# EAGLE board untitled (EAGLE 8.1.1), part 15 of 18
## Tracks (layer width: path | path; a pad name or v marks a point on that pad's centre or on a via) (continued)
S$15152 (continued)
  Bottom 0: 49.1,139.71 49.1,139.4
S$15153
  Bottom 0: 49.1,139.4 49.17,139.18
S$15154
  Bottom 0: 146.37,139.57 146.33,139.85
S$15155
  Bottom 0: 146.33,139.85 146.2,140.13
S$15156
  Bottom 0: 146.2,140.13 145.99,140.34
S$15157
  Bottom 0: 145.99,140.34 145.73,140.5
S$15158
  Bottom 0: 145.73,140.5 145.44,140.56
S$15159
  Bottom 0: 145.44,140.56 145.13,140.54
S$15160
  Bottom 0: 145.13,140.54 144.85,140.43
S$15161
  Bottom 0: 144.85,140.43 144.61,140.24
S$15162
  Bottom 0: 144.61,140.24 144.44,140
S$15163
  Bottom 0: 144.44,140 144.36,139.74
S$15164
  Bottom 0: 144.36,139.74 137.85,139.74
S$15165
  Bottom 0: 137.85,139.74 138.05,139.97
S$15166
  Bottom 0: 138.05,139.97 138.19,140.27
S$15167
  Bottom 0: 138.19,140.27 138.24,140.59
S$15168
  Bottom 0: 138.24,140.59 138.19,140.91
S$15169
  Bottom 0: 138.19,140.91 138.05,141.21
S$15170
  Bottom 0: 138.05,141.21 137.84,141.45
S$15171
  Bottom 0: 137.84,141.45 137.66,141.57
S$15172
  Bottom 0: 137.66,141.57 137.66,145.11
S$15173
  Bottom 0: 137.66,145.11 146.76,154.22
S$15174
  Bottom 0: 146.76,154.22 148.03,155.48
S$15175
  Bottom 0: 148.03,155.48 148,155.43
S$15176
  Bottom 0: 148,155.43 147.87,155.01
S$15177
  Bottom 0: 147.87,155.01 147.83,154.56
S$15178
  Bottom 0: 147.83,154.56 147.87,154.11
S$15179
  Bottom 0: 147.87,154.11 148,153.68
S$15180
  Bottom 0: 148,153.68 148.21,153.29
S$15181
  Bottom 0: 148.21,153.29 148.5,152.94
S$15182
  Bottom 0: 148.5,152.94 148.84,152.66
S$15183
  Bottom 0: 148.84,152.66 149.24,152.45
S$15184
  Bottom 0: 149.24,152.45 149.67,152.32
S$15185
  Bottom 0: 149.67,152.32 150.11,152.27
S$15186
  Bottom 0: 150.11,152.27 150.56,152.32
S$15187
  Bottom 0: 150.56,152.32 150.86,152.41
S$15188
  Bottom 0: 150.86,152.41 149.85,151.4
S$15189
  Bottom 0: 149.85,151.4 149.8,151.34
S$15190
  Bottom 0: 149.8,151.34 149.77,151.29
S$15191
  Bottom 0: 149.77,151.29 149.74,151.22
S$15192
  Bottom 0: 149.74,151.22 149.72,151.16
S$15193
  Bottom 0: 149.72,151.16 149.72,151.08
S$15194
  Bottom 0: 149.72,151.08 149.72,148.84
S$15195
  Bottom 0: 149.72,148.84 147.34,146.47
S$15196
  Bottom 0: 147.34,146.47 147.31,146.41
S$15197
  Bottom 0: 147.31,146.41 147.26,146.35
S$15198
  Bottom 0: 147.26,146.35 147.24,146.29
S$15199
  Bottom 0: 147.24,146.29 147.22,146.22
S$15200
  Bottom 0: 147.22,146.22 147.22,146.15
S$15201
  Bottom 0: 147.22,146.15 147.22,140.42
S$15202
  Bottom 0: 147.22,140.42 146.37,139.57
S$15203
  Bottom 0: 139.57,142.66 139.89,142.68
S$15204
  Bottom 0: 139.89,142.68 140.2,142.78
S$15205
  Bottom 0: 140.2,142.78 140.46,142.97
S$15206
  Bottom 0: 140.46,142.97 140.67,143.23
S$15207
  Bottom 0: 140.67,143.23 140.8,143.52
S$15208
  Bottom 0: 140.8,143.52 140.84,143.84
S$15209
  Bottom 0: 140.84,143.84 140.8,144.16
S$15210
  Bottom 0: 140.8,144.16 140.67,144.47
S$15211
  Bottom 0: 140.67,144.47 140.46,144.72
S$15212
  Bottom 0: 140.46,144.72 140.2,144.91
S$15213
  Bottom 0: 140.2,144.91 139.89,145.01
S$15214
  Bottom 0: 139.89,145.01 139.57,145.03
S$15215
  Bottom 0: 139.57,145.03 139.25,144.97
S$15216
  Bottom 0: 139.25,144.97 138.96,144.82
S$15217
  Bottom 0: 138.96,144.82 138.72,144.6
S$15218
  Bottom 0: 138.72,144.6 138.55,144.32
S$15219
  Bottom 0: 138.55,144.32 138.47,144.01
S$15220
  Bottom 0: 138.47,144.01 138.47,143.68
S$15221
  Bottom 0: 138.47,143.68 138.55,143.37
S$15222
  Bottom 0: 138.55,143.37 138.72,143.09
S$15223
  Bottom 0: 138.72,143.09 138.96,142.87
S$15224
  Bottom 0: 138.96,142.87 139.25,142.72
S$15225
  Bottom 0: 139.25,142.72 139.57,142.66
S$15226
  Bottom 0: 147.66,148.09 148.01,148.15
S$15227
  Bottom 0: 148.01,148.15 148.32,148.3
S$15228
  Bottom 0: 148.32,148.3 148.59,148.52
S$15229
  Bottom 0: 148.59,148.52 148.8,148.81
S$15230
  Bottom 0: 148.8,148.81 148.93,149.13
S$15231
  Bottom 0: 148.93,149.13 148.97,149.48
S$15232
  Bottom 0: 148.97,149.48 148.93,149.82
S$15233
  Bottom 0: 148.93,149.82 148.8,150.15
S$15234
  Bottom 0: 148.8,150.15 148.59,150.43
S$15235
  Bottom 0: 148.59,150.43 148.32,150.66
S$15236
  Bottom 0: 148.32,150.66 148.01,150.81
S$15237
  Bottom 0: 148.01,150.81 147.66,150.87
S$15238
  Bottom 0: 147.66,150.87 147.31,150.85
S$15239
  Bottom 0: 147.31,150.85 146.98,150.74
S$15240
  Bottom 0: 146.98,150.74 146.69,150.56
S$15241
  Bottom 0: 146.69,150.56 146.44,150.3
S$15242
  Bottom 0: 146.44,150.3 146.27,149.99
S$15243
  Bottom 0: 146.27,149.99 146.19,149.65
S$15244
  Bottom 0: 146.19,149.65 146.19,149.3
S$15245
  Bottom 0: 146.19,149.3 146.27,148.97
S$15246
  Bottom 0: 146.27,148.97 146.44,148.66
S$15247
  Bottom 0: 146.44,148.66 146.69,148.4
S$15248
  Bottom 0: 146.69,148.4 146.98,148.21
S$15249
  Bottom 0: 146.98,148.21 147.31,148.11
S$15250
  Bottom 0: 147.31,148.11 147.66,148.09
S$15251
  Bottom 0: 59.5,139.69 59.5,141.48
S$15252
  Bottom 0: 59.5,141.48 59.49,141.55
S$15253
  Bottom 0: 59.49,141.55 59.45,141.62
S$15254
  Bottom 0: 59.45,141.62 59.4,141.68
S$15255
  Bottom 0: 59.4,141.68 59.32,141.72
S$15256
  Bottom 0: 59.32,141.72 59.25,141.73
S$15257
  Bottom 0: 59.25,141.73 58.8,141.73
S$15258
  Bottom 0: 58.8,141.73 58.8,141.86
S$15259
  Bottom 0: 58.8,141.86 58.74,142.08
S$15260
  Bottom 0: 58.74,142.08 58.58,142.24
S$15261
  Bottom 0: 58.58,142.24 58.36,142.3
S$15262
  Bottom 0: 58.36,142.3 57.99,142.3
S$15263
  Bottom 0: 57.99,142.3 56.91,143.38
S$15264
  Bottom 0: 56.91,143.38 56.97,143.52
S$15265
  Bottom 0: 56.97,143.52 57.02,143.84
S$15266
  Bottom 0: 57.02,143.84 56.97,144.16
S$15267
  Bottom 0: 56.97,144.16 56.84,144.46
S$15268
  Bottom 0: 56.84,144.46 56.64,144.71
S$15269
  Bottom 0: 56.64,144.71 56.57,144.76
S$15270
  Bottom 0: 56.57,144.76 61.72,144.76
S$15271
  Bottom 0: 61.72,144.76 62.3,144.18
S$15272
  Bottom 0: 62.3,144.18 62.26,144
S$15273
  Bottom 0: 62.26,144 62.26,143.68
S$15274
  Bottom 0: 62.26,143.68 62.35,143.36
S$15275
  Bottom 0: 62.35,143.36 62.52,143.09
S$15276
  Bottom 0: 62.52,143.09 62.75,142.87
S$15277
  Bottom 0: 62.75,142.87 63.04,142.72
S$15278
  Bottom 0: 63.04,142.72 63.36,142.65
S$15279
  Bottom 0: 63.36,142.65 63.69,142.67
S$15280
  Bottom 0: 63.69,142.67 63.99,142.78
S$15281
  Bottom 0: 63.99,142.78 64.26,142.97
S$15282
  Bottom 0: 64.26,142.97 64.46,143.22
S$15283
  Bottom 0: 64.46,143.22 64.49,143.27
S$15284
  Bottom 0: 64.49,143.27 66.41,143.27
S$15285
  Bottom 0: 66.41,143.27 69.13,140.56
S$15286
  Bottom 0: 69.13,140.56 68.92,140.54
S$15287
  Bottom 0: 68.92,140.54 68.65,140.43
S$15288
  Bottom 0: 68.65,140.43 68.41,140.24
S$15289
  Bottom 0: 68.41,140.24 68.24,140
S$15290
  Bottom 0: 68.24,140 68.15,139.71
S$15291
  Bottom 0: 68.15,139.71 68.15,139.69
S$15292
  Bottom 0: 68.15,139.69 61.59,139.69
S$15293
  Bottom 0: 61.59,139.69 61.65,139.72
S$15294
  Bottom 0: 61.65,139.72 61.86,139.97
S$15295
  Bottom 0: 61.86,139.97 62,140.27
S$15296
  Bottom 0: 62,140.27 62.04,140.59
S$15297
  Bottom 0: 62.04,140.59 62,140.91
S$15298
  Bottom 0: 62,140.91 61.86,141.21
S$15299
  Bottom 0: 61.86,141.21 61.65,141.45
S$15300
  Bottom 0: 61.65,141.45 61.37,141.63
S$15301
  Bottom 0: 61.37,141.63 61.06,141.72
S$15302
  Bottom 0: 61.06,141.72 60.74,141.72
S$15303
  Bottom 0: 60.74,141.72 60.42,141.63
S$15304
  Bottom 0: 60.42,141.63 60.15,141.45
S$15305
  Bottom 0: 60.15,141.45 59.94,141.21
S$15306
  Bottom 0: 59.94,141.21 59.8,140.91
S$15307
  Bottom 0: 59.8,140.91 59.76,140.59
S$15308
  Bottom 0: 59.76,140.59 59.8,140.27
S$15309
  Bottom 0: 59.8,140.27 59.94,139.97
S$15310
  Bottom 0: 59.94,139.97 60.15,139.72
S$15311
  Bottom 0: 60.15,139.72 60.21,139.69
S$15312
  Bottom 0: 60.21,139.69 59.5,139.69
S$15313
  Bottom 0: 154.75,140 154.75,141.48
S$15314
  Bottom 0: 154.75,141.48 154.74,141.55
S$15315
  Bottom 0: 154.74,141.55 154.7,141.62
S$15316
  Bottom 0: 154.7,141.62 154.64,141.68
S$15317
  Bottom 0: 154.64,141.68 154.57,141.72
S$15318
  Bottom 0: 154.57,141.72 154.49,141.73
S$15319
  Bottom 0: 154.49,141.73 154.05,141.73
S$15320
  Bottom 0: 154.05,141.73 154.05,141.86
S$15321
  Bottom 0: 154.05,141.86 153.99,142.08
S$15322
  Bottom 0: 153.99,142.08 153.82,142.24
S$15323
  Bottom 0: 153.82,142.24 153.6,142.3
S$15324
  Bottom 0: 153.6,142.3 153.26,142.3
S$15325
  Bottom 0: 153.26,142.3 152.17,143.39
S$15326
  Bottom 0: 152.17,143.39 152.23,143.52
S$15327
  Bottom 0: 152.23,143.52 152.28,143.84
S$15328
  Bottom 0: 152.28,143.84 152.23,144.16
S$15329
  Bottom 0: 152.23,144.16 152.1,144.47
S$15330
  Bottom 0: 152.1,144.47 151.9,144.72
S$15331
  Bottom 0: 151.9,144.72 151.63,144.91
S$15332
  Bottom 0: 151.63,144.91 151.33,145.01
S$15333
  Bottom 0: 151.33,145.01 151,145.03
S$15334
  Bottom 0: 151,145.03 150.92,145.02
S$15335
  Bottom 0: 150.92,145.02 157.26,151.36
S$15336
  Bottom 0: 157.26,151.36 157.66,151.36
S$15337
  Bottom 0: 157.66,151.36 157.73,151.36
S$15338
  Bottom 0: 157.73,151.36 157.79,151.38
S$15339
  Bottom 0: 157.79,151.38 157.86,151.4
S$15340
  Bottom 0: 157.86,151.4 157.92,151.44
S$15341
  Bottom 0: 157.92,151.44 157.97,151.49
S$15342
  Bottom 0: 157.97,151.49 158.18,151.68
S$15343
  Bottom 0: 158.18,151.68 158.21,151.68
S$15344
  Bottom 0: 158.21,151.68 158.28,151.67
S$15345
  Bottom 0: 158.28,151.67 158.91,151.67
S$15346
  Bottom 0: 158.91,151.67 158.74,151.43
S$15347
  Bottom 0: 158.74,151.43 158.65,151.13
S$15348
  Bottom 0: 158.65,151.13 158.65,150.83
S$15349
  Bottom 0: 158.65,150.83 158.74,150.54
S$15350
  Bottom 0: 158.74,150.54 158.91,150.29
S$15351
  Bottom 0: 158.91,150.29 159.14,150.1
S$15352
  Bottom 0: 159.14,150.1 159.43,149.99
S$15353
  Bottom 0: 159.43,149.99 159.73,149.97
S$15354
  Bottom 0: 159.73,149.97 160.03,150.04
S$15355
  Bottom 0: 160.03,150.04 160.29,150.19
S$15356
  Bottom 0: 160.29,150.19 160.49,150.41
S$15357
  Bottom 0: 160.49,150.41 160.62,150.68
S$15358
  Bottom 0: 160.62,150.68 160.67,150.98
S$15359
  Bottom 0: 160.67,150.98 160.62,151.28
S$15360
  Bottom 0: 160.62,151.28 160.49,151.56
S$15361
  Bottom 0: 160.49,151.56 160.39,151.67
S$15362
  Bottom 0: 160.39,151.67 170.46,151.67
S$15363
  Bottom 0: 170.46,151.67 170.53,151.68
S$15364
  Bottom 0: 170.53,151.68 170.6,151.69
S$15365
  Bottom 0: 170.6,151.69 170.66,151.72
S$15366
  Bottom 0: 170.66,151.72 170.72,151.76
S$15367
  Bottom 0: 170.72,151.76 170.77,151.8
S$15368
  Bottom 0: 170.77,151.8 172.09,153.12
S$15369
  Bottom 0: 172.09,153.12 172.13,153.12
S$15370
  Bottom 0: 172.13,153.12 172.09,153.1
S$15371
  Bottom 0: 172.09,153.1 171.85,152.84
S$15372
  Bottom 0: 171.85,152.84 171.67,152.53
S$15373
  Bottom 0: 171.67,152.53 171.59,152.19
S$15374
  Bottom 0: 171.59,152.19 171.59,151.84
S$15375
  Bottom 0: 171.59,151.84 171.67,151.51
S$15376
  Bottom 0: 171.67,151.51 171.73,151.4
S$15377
  Bottom 0: 171.73,151.4 168.6,148.28
S$15378
  Bottom 0: 168.6,148.28 167.33,148.28
S$15379
  Bottom 0: 167.33,148.28 167.37,148.3
S$15380
  Bottom 0: 167.37,148.3 167.64,148.52
S$15381
  Bottom 0: 167.64,148.52 167.85,148.81
S$15382
  Bottom 0: 167.85,148.81 167.97,149.13
S$15383
  Bottom 0: 167.97,149.13 168.02,149.48
S$15384
  Bottom 0: 168.02,149.48 167.97,149.82
S$15385
  Bottom 0: 167.97,149.82 167.85,150.15
S$15386
  Bottom 0: 167.85,150.15 167.64,150.43
S$15387
  Bottom 0: 167.64,150.43 167.37,150.66
S$15388
  Bottom 0: 167.37,150.66 167.06,150.81
S$15389
  Bottom 0: 167.06,150.81 166.71,150.87
S$15390
  Bottom 0: 166.71,150.87 166.36,150.85
S$15391
  Bottom 0: 166.36,150.85 166.03,150.74
S$15392
  Bottom 0: 166.03,150.74 165.74,150.56
S$15393
  Bottom 0: 165.74,150.56 165.49,150.3
S$15394
  Bottom 0: 165.49,150.3 165.32,149.99
S$15395
  Bottom 0: 165.32,149.99 165.24,149.65
S$15396
  Bottom 0: 165.24,149.65 165.24,149.3
S$15397
  Bottom 0: 165.24,149.3 165.32,148.97
S$15398
  Bottom 0: 165.32,148.97 165.49,148.66
S$15399
  Bottom 0: 165.49,148.66 165.74,148.4
S$15400
  Bottom 0: 165.74,148.4 165.93,148.28
S$15401
  Bottom 0: 165.93,148.28 155.93,148.28
S$15402
  Bottom 0: 155.93,148.28 155.86,148.28
S$15403
  Bottom 0: 155.86,148.28 155.79,148.26
S$15404
  Bottom 0: 155.79,148.26 155.73,148.23
S$15405
  Bottom 0: 155.73,148.23 155.67,148.19
S$15406
  Bottom 0: 155.67,148.19 155.62,148.15
S$15407
  Bottom 0: 155.62,148.15 153.85,146.39
S$15408
  Bottom 0: 153.85,146.39 153.81,146.33
S$15409
  Bottom 0: 153.81,146.33 153.77,146.28
S$15410
  Bottom 0: 153.77,146.28 153.74,146.21
S$15411
  Bottom 0: 153.74,146.21 153.73,146.15
S$15412
  Bottom 0: 153.73,146.15 153.72,146.07
S$15413
  Bottom 0: 153.72,146.07 153.72,144.78
S$15414
  Bottom 0: 153.72,144.78 153.73,144.71
S$15415
  Bottom 0: 153.73,144.71 153.74,144.64
S$15416
  Bottom 0: 153.74,144.64 153.77,144.58
S$15417
  Bottom 0: 153.77,144.58 153.81,144.52
S$15418
  Bottom 0: 153.81,144.52 153.85,144.47
S$15419
  Bottom 0: 153.85,144.47 156.8,141.51
S$15420
  Bottom 0: 156.8,141.51 156.62,141.63
S$15421
  Bottom 0: 156.62,141.63 156.31,141.72
S$15422
  Bottom 0: 156.31,141.72 155.98,141.72
S$15423
  Bottom 0: 155.98,141.72 155.67,141.63
S$15424
  Bottom 0: 155.67,141.63 155.4,141.45
S$15425
  Bottom 0: 155.4,141.45 155.18,141.21
S$15426
  Bottom 0: 155.18,141.21 155.04,140.91
S$15427
  Bottom 0: 155.04,140.91 155,140.59
S$15428
  Bottom 0: 155,140.59 155.04,140.29
S$15429
  Bottom 0: 155.04,140.29 154.75,140
S$15430
  Bottom 0: 240.79,142.26 240.78,142.27
S$15431
  Bottom 0: 240.78,142.27 240.72,142.29
S$15432
  Bottom 0: 240.72,142.29 240.65,142.29
S$15433
  Bottom 0: 240.65,142.29 223.56,142.29
S$15434
  Bottom 0: 223.56,142.29 207.94,157.9
S$15435
  Bottom 0: 207.94,157.9 211.02,157.9
S$15436
  Bottom 0: 211.02,157.9 216.95,151.98
S$15437
  Bottom 0: 216.95,151.98 216.88,151.99
S$15438
  Bottom 0: 216.88,151.99 216.58,151.97
S$15439
  Bottom 0: 216.58,151.97 216.3,151.86
S$15440
  Bottom 0: 216.3,151.86 216.06,151.67
S$15441
  Bottom 0: 216.06,151.67 215.89,151.43
S$15442
  Bottom 0: 215.89,151.43 215.8,151.13
S$15443
  Bottom 0: 215.8,151.13 215.8,150.83
S$15444
  Bottom 0: 215.8,150.83 215.89,150.54
S$15445
  Bottom 0: 215.89,150.54 216.06,150.29
S$15446
  Bottom 0: 216.06,150.29 216.3,150.1
S$15447
  Bottom 0: 216.3,150.1 216.58,149.99
S$15448
  Bottom 0: 216.58,149.99 216.88,149.97
S$15449
  Bottom 0: 216.88,149.97 217.18,150.04
S$15450
  Bottom 0: 217.18,150.04 217.44,150.19
S$15451
  Bottom 0: 217.44,150.19 217.64,150.41
S$15452
  Bottom 0: 217.64,150.41 217.71,150.54
S$15453
  Bottom 0: 217.71,150.54 222.08,150.54
S$15454
  Bottom 0: 222.08,150.54 222.53,150.09
S$15455
  Bottom 0: 222.53,150.09 222.47,149.99
S$15456
  Bottom 0: 222.47,149.99 222.39,149.65
S$15457
  Bottom 0: 222.39,149.65 222.39,149.3
S$15458
  Bottom 0: 222.39,149.3 222.47,148.97
S$15459
  Bottom 0: 222.47,148.97 222.65,148.66
S$15460
  Bottom 0: 222.65,148.66 222.88,148.4
S$15461
  Bottom 0: 222.88,148.4 223.18,148.21
S$15462
  Bottom 0: 223.18,148.21 223.51,148.11
S$15463
  Bottom 0: 223.51,148.11 223.86,148.09
S$15464
  Bottom 0: 223.86,148.09 224.21,148.15
S$15465
  Bottom 0: 224.21,148.15 224.52,148.3
S$15466
  Bottom 0: 224.52,148.3 224.79,148.52
S$15467
  Bottom 0: 224.79,148.52 225,148.81
S$15468
  Bottom 0: 225,148.81 225.12,149.13
S$15469
  Bottom 0: 225.12,149.13 225.17,149.48
S$15470
  Bottom 0: 225.17,149.48 225.12,149.82
S$15471
  Bottom 0: 225.12,149.82 225,150.15
S$15472
  Bottom 0: 225,150.15 224.79,150.43
S$15473
  Bottom 0: 224.79,150.43 224.52,150.66
S$15474
  Bottom 0: 224.52,150.66 224.21,150.81
S$15475
  Bottom 0: 224.21,150.81 223.86,150.87
S$15476
  Bottom 0: 223.86,150.87 223.51,150.85
S$15477
  Bottom 0: 223.51,150.85 223.18,150.74
S$15478
  Bottom 0: 223.18,150.74 223.15,150.72
S$15479
  Bottom 0: 223.15,150.72 222.57,151.3
S$15480
  Bottom 0: 222.57,151.3 222.52,151.34
S$15481
  Bottom 0: 222.52,151.34 222.46,151.38
S$15482
  Bottom 0: 222.46,151.38 222.4,151.4
S$15483
  Bottom 0: 222.4,151.4 222.33,151.42
S$15484
  Bottom 0: 222.33,151.42 222.26,151.43
S$15485
  Bottom 0: 222.26,151.43 217.71,151.43
S$15486
  Bottom 0: 217.71,151.43 217.64,151.56
S$15487
  Bottom 0: 217.64,151.56 217.62,151.58
S$15488
  Bottom 0: 217.62,151.58 228.8,151.58
S$15489
  Bottom 0: 228.8,151.58 228.82,151.51
S$15490
  Bottom 0: 228.82,151.51 229,151.2
S$15491
  Bottom 0: 229,151.2 229.24,150.94
S$15492
  Bottom 0: 229.24,150.94 229.53,150.75
S$15493
  Bottom 0: 229.53,150.75 229.86,150.65
S$15494
  Bottom 0: 229.86,150.65 230.21,150.63
S$15495
  Bottom 0: 230.21,150.63 230.56,150.69
S$15496
  Bottom 0: 230.56,150.69 230.87,150.84
S$15497
  Bottom 0: 230.87,150.84 231.14,151.06
S$15498
  Bottom 0: 231.14,151.06 231.35,151.35
S$15499
  Bottom 0: 231.35,151.35 231.44,151.58
S$15500
  Bottom 0: 231.44,151.58 231.48,151.58
S$15501
  Bottom 0: 231.48,151.58 240.79,142.26
S$15502
  Bottom 0: 227.21,142.65 227.53,142.67
S$15503
  Bottom 0: 227.53,142.67 227.84,142.78
S$15504
  Bottom 0: 227.84,142.78 228.1,142.97
S$15505
  Bottom 0: 228.1,142.97 228.31,143.22
S$15506
  Bottom 0: 228.31,143.22 228.44,143.52
S$15507
  Bottom 0: 228.44,143.52 228.48,143.84
S$15508
  Bottom 0: 228.48,143.84 228.44,144.16
S$15509
  Bottom 0: 228.44,144.16 228.31,144.46
S$15510
  Bottom 0: 228.31,144.46 228.1,144.71
S$15511
  Bottom 0: 228.1,144.71 227.84,144.9
S$15512
  Bottom 0: 227.84,144.9 227.53,145.01
S$15513
  Bottom 0: 227.53,145.01 227.21,145.03
S$15514
  Bottom 0: 227.21,145.03 226.89,144.96
S$15515
  Bottom 0: 226.89,144.96 226.6,144.82
S$15516
  Bottom 0: 226.6,144.82 226.37,144.59
S$15517
  Bottom 0: 226.37,144.59 226.19,144.32
S$15518
  Bottom 0: 226.19,144.32 226.11,144
S$15519
  Bottom 0: 226.11,144 226.11,143.68
S$15520
  Bottom 0: 226.11,143.68 226.19,143.36
S$15521
  Bottom 0: 226.19,143.36 226.37,143.09
S$15522
  Bottom 0: 226.37,143.09 226.6,142.87
S$15523
  Bottom 0: 226.6,142.87 226.89,142.72
S$15524
  Bottom 0: 226.89,142.72 227.21,142.65
S$15525
  Bottom 0: 234.83,142.65 235.15,142.67
S$15526
  Bottom 0: 235.15,142.67 235.46,142.78
S$15527
  Bottom 0: 235.46,142.78 235.72,142.97
S$15528
  Bottom 0: 235.72,142.97 235.93,143.22
S$15529
  Bottom 0: 235.93,143.22 236.06,143.52
S$15530
  Bottom 0: 236.06,143.52 236.1,143.84
S$15531
  Bottom 0: 236.1,143.84 236.06,144.16
S$15532
  Bottom 0: 236.06,144.16 235.93,144.46
S$15533
  Bottom 0: 235.93,144.46 235.72,144.71
S$15534
  Bottom 0: 235.72,144.71 235.46,144.9
S$15535
  Bottom 0: 235.46,144.9 235.15,145.01
S$15536
  Bottom 0: 235.15,145.01 234.83,145.03
S$15537
  Bottom 0: 234.83,145.03 234.51,144.96
S$15538
  Bottom 0: 234.51,144.96 234.22,144.82
S$15539
  Bottom 0: 234.22,144.82 233.99,144.59
S$15540
  Bottom 0: 233.99,144.59 233.81,144.32
S$15541
  Bottom 0: 233.81,144.32 233.73,144
S$15542
  Bottom 0: 233.73,144 233.73,143.68
S$15543
  Bottom 0: 233.73,143.68 233.81,143.36
S$15544
  Bottom 0: 233.81,143.36 233.99,143.09
S$15545
  Bottom 0: 233.99,143.09 234.22,142.87
S$15546
  Bottom 0: 234.22,142.87 234.51,142.72
S$15547
  Bottom 0: 234.51,142.72 234.83,142.65
S$15548
  Bottom 0: 103.41,142.78 102.69,143.5
S$15549
  Bottom 0: 102.69,143.5 102.69,143.52
S$15550
  Bottom 0: 102.69,143.52 102.74,143.84
S$15551
  Bottom 0: 102.74,143.84 102.69,144.16
S$15552
  Bottom 0: 102.69,144.16 102.69,144.18
S$15553
  Bottom 0: 102.69,144.18 104.18,145.67
S$15554
  Bottom 0: 104.18,145.67 104.24,145.74
S$15555
  Bottom 0: 104.24,145.74 104.28,145.81
S$15556
  Bottom 0: 104.28,145.81 104.32,145.89
S$15557
  Bottom 0: 104.32,145.89 104.34,145.98
S$15558
  Bottom 0: 104.34,145.98 104.34,146.07
S$15559
  Bottom 0: 104.34,146.07 104.34,162.5
S$15560
  Bottom 0: 104.34,162.5 104.65,162.8
S$15561
  Bottom 0: 104.65,162.8 104.65,162.75
S$15562
  Bottom 0: 104.65,162.75 104.74,162.52
S$15563
  Bottom 0: 104.74,162.52 104.91,162.33
S$15564
  Bottom 0: 104.91,162.33 105.13,162.22
S$15565
  Bottom 0: 105.13,162.22 105.16,162.22
S$15566
  Bottom 0: 105.16,162.22 109.98,157.4
S$15567
  Bottom 0: 109.98,157.4 110.04,157.36
S$15568
  Bottom 0: 110.04,157.36 110.1,157.32
S$15569
  Bottom 0: 110.1,157.32 110.16,157.29
S$15570
  Bottom 0: 110.16,157.29 110.23,157.28
S$15571
  Bottom 0: 110.23,157.28 110.3,157.27
S$15572
  Bottom 0: 110.3,157.27 112.2,157.27
S$15573
  Bottom 0: 112.2,157.27 112.76,156.71
S$15574
  Bottom 0: 112.76,156.71 112.46,156.8
S$15575
  Bottom 0: 112.46,156.8 112.01,156.84
S$15576
  Bottom 0: 112.01,156.84 111.57,156.8
S$15577
  Bottom 0: 111.57,156.8 111.14,156.67
S$15578
  Bottom 0: 111.14,156.67 110.74,156.46
S$15579
  Bottom 0: 110.74,156.46 110.4,156.17
S$15580
  Bottom 0: 110.4,156.17 110.11,155.83
S$15581
  Bottom 0: 110.11,155.83 109.9,155.43
S$15582
  Bottom 0: 109.9,155.43 109.77,155.01
S$15583
  Bottom 0: 109.77,155.01 109.73,154.56
S$15584
  Bottom 0: 109.73,154.56 109.77,154.11
S$15585
  Bottom 0: 109.77,154.11 109.9,153.68
S$15586
  Bottom 0: 109.9,153.68 110.11,153.29
S$15587
  Bottom 0: 110.11,153.29 110.4,152.94
S$15588
  Bottom 0: 110.4,152.94 110.74,152.66
S$15589
  Bottom 0: 110.74,152.66 111.14,152.45
S$15590
  Bottom 0: 111.14,152.45 111.57,152.32
S$15591
  Bottom 0: 111.57,152.32 112.01,152.27
S$15592
  Bottom 0: 112.01,152.27 112.46,152.32
S$15593
  Bottom 0: 112.46,152.32 112.89,152.45
S$15594
  Bottom 0: 112.89,152.45 113.28,152.66
S$15595
  Bottom 0: 113.28,152.66 113.63,152.94
S$15596
  Bottom 0: 113.63,152.94 113.91,153.29
S$15597
  Bottom 0: 113.91,153.29 114.13,153.68
S$15598
  Bottom 0: 114.13,153.68 114.25,154.11
S$15599
  Bottom 0: 114.25,154.11 114.3,154.56
S$15600
  Bottom 0: 114.3,154.56 114.25,155.01
S$15601
  Bottom 0: 114.25,155.01 114.16,155.31
S$15602
  Bottom 0: 114.16,155.31 115.38,154.09
S$15603
  Bottom 0: 115.38,154.09 115.38,153.34
S$15604
  Bottom 0: 115.38,153.34 115.23,153.28
S$15605
  Bottom 0: 115.23,153.28 114.94,153.1
S$15606
  Bottom 0: 114.94,153.1 114.69,152.84
S$15607
  Bottom 0: 114.69,152.84 114.52,152.53
S$15608
  Bottom 0: 114.52,152.53 114.44,152.19
S$15609
  Bottom 0: 114.44,152.19 114.44,151.84
S$15610
  Bottom 0: 114.44,151.84 114.52,151.51
S$15611
  Bottom 0: 114.52,151.51 114.69,151.2
S$15612
  Bottom 0: 114.69,151.2 114.94,150.94
S$15613
  Bottom 0: 114.94,150.94 115.23,150.75
S$15614
  Bottom 0: 115.23,150.75 115.56,150.65
S$15615
  Bottom 0: 115.56,150.65 115.91,150.63
S$15616
  Bottom 0: 115.91,150.63 116.26,150.69
S$15617
  Bottom 0: 116.26,150.69 116.44,150.78
S$15618
  Bottom 0: 116.44,150.78 121.51,145.7
S$15619
  Bottom 0: 121.51,145.7 121.51,144.6
S$15620
  Bottom 0: 121.51,144.6 121.41,144.72
S$15621
  Bottom 0: 121.41,144.72 121.15,144.91
S$15622
  Bottom 0: 121.15,144.91 120.84,145.01
S$15623
  Bottom 0: 120.84,145.01 120.52,145.03
S$15624
  Bottom 0: 120.52,145.03 120.2,144.97
S$15625
  Bottom 0: 120.2,144.97 119.91,144.82
S$15626
  Bottom 0: 119.91,144.82 119.67,144.6
S$15627
  Bottom 0: 119.67,144.6 119.5,144.32
S$15628
  Bottom 0: 119.5,144.32 119.42,144.01
S$15629
  Bottom 0: 119.42,144.01 119.42,143.68
S$15630
  Bottom 0: 119.42,143.68 119.46,143.51
S$15631
  Bottom 0: 119.46,143.51 118.72,142.78
S$15632
  Bottom 0: 118.72,142.78 113.51,142.78
S$15633
  Bottom 0: 113.51,142.78 113.53,142.78
S$15634
  Bottom 0: 113.53,142.78 113.79,142.97
S$15635
  Bottom 0: 113.79,142.97 114,143.23
S$15636
  Bottom 0: 114,143.23 114.13,143.52
S$15637
  Bottom 0: 114.13,143.52 114.17,143.84
S$15638
  Bottom 0: 114.17,143.84 114.13,144.16
S$15639
  Bottom 0: 114.13,144.16 114,144.47
S$15640
  Bottom 0: 114,144.47 113.79,144.72
S$15641
  Bottom 0: 113.79,144.72 113.53,144.91
S$15642
  Bottom 0: 113.53,144.91 113.22,145.01
S$15643
  Bottom 0: 113.22,145.01 112.9,145.03
S$15644
  Bottom 0: 112.9,145.03 112.58,144.97
S$15645
  Bottom 0: 112.58,144.97 112.29,144.82
S$15646
  Bottom 0: 112.29,144.82 112.06,144.6
S$15647
  Bottom 0: 112.06,144.6 111.88,144.32
S$15648
  Bottom 0: 111.88,144.32 111.8,144.01
S$15649
  Bottom 0: 111.8,144.01 111.8,143.68
S$15650
  Bottom 0: 111.8,143.68 111.88,143.37
S$15651
  Bottom 0: 111.88,143.37 112.06,143.09
S$15652
  Bottom 0: 112.06,143.09 112.29,142.87
S$15653
  Bottom 0: 112.29,142.87 112.47,142.78
S$15654
  Bottom 0: 112.47,142.78 103.41,142.78
S$15655
  Bottom 0: 109.56,148.09 109.91,148.15
S$15656
  Bottom 0: 109.91,148.15 110.22,148.3
S$15657
  Bottom 0: 110.22,148.3 110.49,148.52
S$15658
  Bottom 0: 110.49,148.52 110.7,148.81
S$15659
  Bottom 0: 110.7,148.81 110.83,149.13
S$15660
  Bottom 0: 110.83,149.13 110.87,149.48
S$15661
  Bottom 0: 110.87,149.48 110.83,149.82
S$15662
  Bottom 0: 110.83,149.82 110.7,150.15
S$15663
  Bottom 0: 110.7,150.15 110.49,150.43
S$15664
  Bottom 0: 110.49,150.43 110.22,150.66
S$15665
  Bottom 0: 110.22,150.66 109.91,150.81
S$15666
  Bottom 0: 109.91,150.81 109.56,150.87
S$15667
  Bottom 0: 109.56,150.87 109.21,150.85
S$15668
  Bottom 0: 109.21,150.85 108.88,150.74
S$15669
  Bottom 0: 108.88,150.74 108.58,150.56
S$15670
  Bottom 0: 108.58,150.56 108.34,150.3
S$15671
  Bottom 0: 108.34,150.3 108.17,149.99
S$15672
  Bottom 0: 108.17,149.99 108.09,149.65
S$15673
  Bottom 0: 108.09,149.65 108.09,149.3
S$15674
  Bottom 0: 108.09,149.3 108.17,148.97
S$15675
  Bottom 0: 108.17,148.97 108.34,148.66
S$15676
  Bottom 0: 108.34,148.66 108.58,148.4
S$15677
  Bottom 0: 108.58,148.4 108.88,148.21
S$15678
  Bottom 0: 108.88,148.21 109.21,148.11
S$15679
  Bottom 0: 109.21,148.11 109.56,148.09
S$15680
  Bottom 0: 261.74,142.83 258.56,146.01
S$15681
  Bottom 0: 258.56,146.01 258.55,146.02
S$15682
  Bottom 0: 258.55,146.02 253.27,151.3
S$15683
  Bottom 0: 253.27,151.3 253.22,151.35
S$15684
  Bottom 0: 253.22,151.35 253.16,151.39
S$15685
  Bottom 0: 253.16,151.39 253.1,151.41
S$15686
  Bottom 0: 253.1,151.41 253.03,151.43
S$15687
  Bottom 0: 253.03,151.43 252.96,151.44
S$15688
  Bottom 0: 252.96,151.44 250.43,151.44
S$15689
  Bottom 0: 250.43,151.44 250.53,151.67
S$15690
  Bottom 0: 250.53,151.67 250.57,152.02
S$15691
  Bottom 0: 250.57,152.02 250.53,152.36
S$15692
  Bottom 0: 250.53,152.36 250.4,152.69
S$15693
  Bottom 0: 250.4,152.69 250.19,152.97
S$15694
  Bottom 0: 250.19,152.97 249.92,153.2
S$15695
  Bottom 0: 249.92,153.2 249.61,153.35
S$15696
  Bottom 0: 249.61,153.35 249.26,153.41
S$15697
  Bottom 0: 249.26,153.41 248.91,153.39
S$15698
  Bottom 0: 248.91,153.39 248.58,153.28
S$15699
  Bottom 0: 248.58,153.28 248.28,153.1
S$15700
  Bottom 0: 248.28,153.1 248.05,152.84
S$15701
  Bottom 0: 248.05,152.84 247.87,152.53
S$15702
  Bottom 0: 247.87,152.53 247.85,152.46
S$15703
  Bottom 0: 247.85,152.46 246.27,152.46
S$15704
  Bottom 0: 246.27,152.46 246.63,152.66
S$15705
  Bottom 0: 246.63,152.66 246.98,152.94
S$15706
  Bottom 0: 246.98,152.94 247.26,153.29
S$15707
  Bottom 0: 247.26,153.29 247.48,153.68
S$15708
  Bottom 0: 247.48,153.68 247.6,154.11
S$15709
  Bottom 0: 247.6,154.11 247.65,154.56
S$15710
  Bottom 0: 247.65,154.56 247.6,155.01
S$15711
  Bottom 0: 247.6,155.01 247.48,155.43
S$15712
  Bottom 0: 247.48,155.43 247.26,155.83
S$15713
  Bottom 0: 247.26,155.83 246.98,156.17
S$15714
  Bottom 0: 246.98,156.17 246.63,156.46
S$15715
  Bottom 0: 246.63,156.46 246.24,156.67
S$15716
  Bottom 0: 246.24,156.67 245.81,156.8
S$15717
  Bottom 0: 245.81,156.8 245.36,156.84
S$15718
  Bottom 0: 245.36,156.84 244.92,156.8
S$15719
  Bottom 0: 244.92,156.8 244.49,156.67
S$15720
  Bottom 0: 244.49,156.67 244.09,156.46
S$15721
  Bottom 0: 244.09,156.46 243.75,156.17
S$15722
  Bottom 0: 243.75,156.17 243.46,155.83
S$15723
  Bottom 0: 243.46,155.83 243.25,155.43
S$15724
  Bottom 0: 243.25,155.43 243.12,155.01
S$15725
  Bottom 0: 243.12,155.01 243.08,154.56
S$15726
  Bottom 0: 243.08,154.56 243.12,154.11
S$15727
  Bottom 0: 243.12,154.11 243.25,153.68
S$15728
  Bottom 0: 243.25,153.68 243.46,153.29
S$15729
  Bottom 0: 243.46,153.29 243.75,152.94
S$15730
  Bottom 0: 243.75,152.94 244.09,152.66
S$15731
  Bottom 0: 244.09,152.66 244.46,152.46
S$15732
  Bottom 0: 244.46,152.46 241.49,152.46
S$15733
  Bottom 0: 241.49,152.46 235.92,158.03
S$15734
  Bottom 0: 235.92,158.03 235.87,158.07
S$15735
  Bottom 0: 235.87,158.07 235.81,158.11
S$15736
  Bottom 0: 235.81,158.11 235.75,158.13
S$15737
  Bottom 0: 235.75,158.13 235.68,158.15
S$15738
  Bottom 0: 235.68,158.15 235.61,158.16
S$15739
  Bottom 0: 235.61,158.16 219.48,158.16
S$15740
  Bottom 0: 219.48,158.16 213.66,163.98
S$15741
  Bottom 0: 213.66,163.98 213.6,164.03
S$15742
  Bottom 0: 213.6,164.03 213.54,164.07
S$15743
  Bottom 0: 213.54,164.07 213.48,164.09
S$15744
  Bottom 0: 213.48,164.09 213.41,164.11
S$15745
  Bottom 0: 213.41,164.11 213.34,164.11
S$15746
  Bottom 0: 213.34,164.11 213.29,164.11
S$15747
  Bottom 0: 213.29,164.11 213.55,164.21
S$15748
  Bottom 0: 213.55,164.21 213.81,164.39
S$15749
  Bottom 0: 213.81,164.39 214.02,164.65
S$15750
  Bottom 0: 214.02,164.65 214.15,164.95
S$15751
  Bottom 0: 214.15,164.95 214.19,165.27
S$15752
  Bottom 0: 214.19,165.27 214.15,165.59
S$15753
  Bottom 0: 214.15,165.59 214.02,165.89
S$15754
  Bottom 0: 214.02,165.89 213.81,166.14
S$15755
  Bottom 0: 213.81,166.14 213.55,166.33
S$15756
  Bottom 0: 213.55,166.33 213.24,166.44
S$15757
  Bottom 0: 213.24,166.44 213.13,166.44
S$15758
  Bottom 0: 213.13,166.44 213.13,167.7
S$15759
  Bottom 0: 213.13,167.7 213.36,167.45
S$15760
  Bottom 0: 213.36,167.45 213.66,167.26
S$15761
  Bottom 0: 213.66,167.26 213.99,167.16
S$15762
  Bottom 0: 213.99,167.16 214.33,167.14
S$15763
  Bottom 0: 214.33,167.14 214.68,167.2
S$15764
  Bottom 0: 214.68,167.2 215,167.35
S$15765
  Bottom 0: 215,167.35 215.26,167.57
S$15766
  Bottom 0: 215.26,167.57 215.47,167.86
S$15767
  Bottom 0: 215.47,167.86 215.6,168.18
S$15768
  Bottom 0: 215.6,168.18 215.65,168.53
S$15769
  Bottom 0: 215.65,168.53 215.6,168.87
S$15770
  Bottom 0: 215.6,168.87 215.47,169.2
S$15771
  Bottom 0: 215.47,169.2 215.26,169.48
S$15772
  Bottom 0: 215.26,169.48 215,169.71
S$15773
  Bottom 0: 215,169.71 214.69,169.85
S$15774
  Bottom 0: 214.69,169.85 214.69,172.71
S$15775
  Bottom 0: 214.69,172.71 214.89,172.34
S$15776
  Bottom 0: 214.89,172.34 215.17,171.99
S$15777
  Bottom 0: 215.17,171.99 215.52,171.71
S$15778
  Bottom 0: 215.52,171.71 215.91,171.5
S$15779
  Bottom 0: 215.91,171.5 216.34,171.37
S$15780
  Bottom 0: 216.34,171.37 216.79,171.32
S$15781
  Bottom 0: 216.79,171.32 217.24,171.37
S$15782
  Bottom 0: 217.24,171.37 217.66,171.5
S$15783
  Bottom 0: 217.66,171.5 218.06,171.71
S$15784
  Bottom 0: 218.06,171.71 218.33,171.93
S$15785
  Bottom 0: 218.33,171.93 218.33,170.44
S$15786
  Bottom 0: 218.33,170.44 218.34,170.35
S$15787
  Bottom 0: 218.34,170.35 218.36,170.26
S$15788
  Bottom 0: 218.36,170.26 218.39,170.18
S$15789
  Bottom 0: 218.39,170.18 218.44,170.1
S$15790
  Bottom 0: 218.44,170.1 218.5,170.04
S$15791
  Bottom 0: 218.5,170.04 227.01,161.52
S$15792
  Bottom 0: 227.01,161.52 227.01,160.62
S$15793
  Bottom 0: 227.01,160.62 226.84,160.5
S$15794
  Bottom 0: 226.84,160.5 226.62,160.26
S$15795
  Bottom 0: 226.62,160.26 226.49,159.96
S$15796
  Bottom 0: 226.49,159.96 226.44,159.64
S$15797
  Bottom 0: 226.44,159.64 226.49,159.32
S$15798
  Bottom 0: 226.49,159.32 226.62,159.02
S$15799
  Bottom 0: 226.62,159.02 226.84,158.78
S$15800
  Bottom 0: 226.84,158.78 227.11,158.6
S$15801
  Bottom 0: 227.11,158.6 227.42,158.51
S$15802
  Bottom 0: 227.42,158.51 227.75,158.51
S$15803
  Bottom 0: 227.75,158.51 228.05,158.6
S$15804
  Bottom 0: 228.05,158.6 228.33,158.78
S$15805
  Bottom 0: 228.33,158.78 228.54,159.02
S$15806
  Bottom 0: 228.54,159.02 228.68,159.32
S$15807
  Bottom 0: 228.68,159.32 228.73,159.64
S$15808
  Bottom 0: 228.73,159.64 228.68,159.96
S$15809
  Bottom 0: 228.68,159.96 228.54,160.26
S$15810
  Bottom 0: 228.54,160.26 228.33,160.5
S$15811
  Bottom 0: 228.33,160.5 228.15,160.62
S$15812
  Bottom 0: 228.15,160.62 228.15,161.76
S$15813
  Bottom 0: 228.15,161.76 228.15,161.85
S$15814
  Bottom 0: 228.15,161.85 228.13,161.94
S$15815
  Bottom 0: 228.13,161.94 228.09,162.02
S$15816
  Bottom 0: 228.09,162.02 228.05,162.09
S$15817
  Bottom 0: 228.05,162.09 227.99,162.16
S$15818
  Bottom 0: 227.99,162.16 220.45,169.69
S$15819
  Bottom 0: 220.45,169.69 220.68,169.68
S$15820
  Bottom 0: 220.68,169.68 221.03,169.74
S$15821
  Bottom 0: 221.03,169.74 221.21,169.82
S$15822
  Bottom 0: 221.21,169.82 222.52,168.51
S$15823
  Bottom 0: 222.52,168.51 222.58,168.47
S$15824
  Bottom 0: 222.58,168.47 222.64,168.43
S$15825
  Bottom 0: 222.64,168.43 222.7,168.4
S$15826
  Bottom 0: 222.7,168.4 222.77,168.39
S$15827
  Bottom 0: 222.77,168.39 222.84,168.38
S$15828
  Bottom 0: 222.84,168.38 225.88,168.38
S$15829
  Bottom 0: 225.88,168.38 230.19,164.07
S$15830
  Bottom 0: 230.19,164.07 230.06,164.08
S$15831
  Bottom 0: 230.06,164.08 229.74,164.02
S$15832
  Bottom 0: 229.74,164.02 229.45,163.87
S$15833
  Bottom 0: 229.45,163.87 229.22,163.65
S$15834
  Bottom 0: 229.22,163.65 229.05,163.37
S$15835
  Bottom 0: 229.05,163.37 228.96,163.06
S$15836
  Bottom 0: 228.96,163.06 228.96,162.73
S$15837
  Bottom 0: 228.96,162.73 229.05,162.42
S$15838
  Bottom 0: 229.05,162.42 229.22,162.14
S$15839
  Bottom 0: 229.22,162.14 229.45,161.92
S$15840
  Bottom 0: 229.45,161.92 229.74,161.77
S$15841
  Bottom 0: 229.74,161.77 230.06,161.71
S$15842
  Bottom 0: 230.06,161.71 230.39,161.73
S$15843
  Bottom 0: 230.39,161.73 230.69,161.83
S$15844
  Bottom 0: 230.69,161.83 230.96,162.02
S$15845
  Bottom 0: 230.96,162.02 231.16,162.28
S$15846
  Bottom 0: 231.16,162.28 231.29,162.57
S$15847
  Bottom 0: 231.29,162.57 231.34,162.89
S$15848
  Bottom 0: 231.34,162.89 231.33,162.93
S$15849
  Bottom 0: 231.33,162.93 236.97,157.29
S$15850
  Bottom 0: 236.97,157.29 237.03,157.25
S$15851
  Bottom 0: 237.03,157.25 237.09,157.21
S$15852
  Bottom 0: 237.09,157.21 237.15,157.19
S$15853
  Bottom 0: 237.15,157.19 237.22,157.17
S$15854
  Bottom 0: 237.22,157.17 237.29,157.16
S$15855
  Bottom 0: 237.29,157.16 246.62,157.16
S$15856
  Bottom 0: 246.62,157.16 252.08,151.7
S$15857
  Bottom 0: 252.08,151.7 252.14,151.66
S$15858
  Bottom 0: 252.14,151.66 252.2,151.62
S$15859
  Bottom 0: 252.2,151.62 252.26,151.6
S$15860
  Bottom 0: 252.26,151.6 252.32,151.58
S$15861
  Bottom 0: 252.32,151.58 252.4,151.58
S$15862
  Bottom 0: 252.4,151.58 271.66,151.58
S$15863
  Bottom 0: 271.66,151.58 271.68,151.51
S$15864
  Bottom 0: 271.68,151.51 271.86,151.2
S$15865
  Bottom 0: 271.86,151.2 272.1,150.94
S$15866
  Bottom 0: 272.1,150.94 272.39,150.75
S$15867
  Bottom 0: 272.39,150.75 272.72,150.65
S$15868
  Bottom 0: 272.72,150.65 273.07,150.63
S$15869
  Bottom 0: 273.07,150.63 273.42,150.69
S$15870
  Bottom 0: 273.42,150.69 273.73,150.84
S$15871
  Bottom 0: 273.73,150.84 274,151.06
S$15872
  Bottom 0: 274,151.06 274.21,151.35
S$15873
  Bottom 0: 274.21,151.35 274.33,151.67
S$15874
  Bottom 0: 274.33,151.67 274.38,152.02
S$15875
  Bottom 0: 274.38,152.02 274.33,152.36
S$15876
  Bottom 0: 274.33,152.36 274.21,152.69
S$15877
  Bottom 0: 274.21,152.69 274,152.97
S$15878
  Bottom 0: 274,152.97 273.73,153.2
S$15879
  Bottom 0: 273.73,153.2 273.42,153.35
S$15880
  Bottom 0: 273.42,153.35 273.07,153.41
S$15881
  Bottom 0: 273.07,153.41 272.72,153.39
S$15882
  Bottom 0: 272.72,153.39 272.39,153.28
S$15883
  Bottom 0: 272.39,153.28 272.1,153.1
S$15884
  Bottom 0: 272.1,153.1 271.86,152.84
S$15885
  Bottom 0: 271.86,152.84 271.68,152.53
S$15886
  Bottom 0: 271.68,152.53 271.66,152.46
S$15887
  Bottom 0: 271.66,152.46 270.08,152.46
S$15888
  Bottom 0: 270.08,152.46 270.44,152.66
S$15889
  Bottom 0: 270.44,152.66 270.79,152.94
S$15890
  Bottom 0: 270.79,152.94 271.07,153.29
S$15891
  Bottom 0: 271.07,153.29 271.29,153.68
S$15892
  Bottom 0: 271.29,153.68 271.41,154.11
S$15893
  Bottom 0: 271.41,154.11 271.46,154.56
S$15894
  Bottom 0: 271.46,154.56 271.41,155.01
S$15895
  Bottom 0: 271.41,155.01 271.29,155.43
S$15896
  Bottom 0: 271.29,155.43 271.07,155.83
S$15897
  Bottom 0: 271.07,155.83 270.79,156.17
S$15898
  Bottom 0: 270.79,156.17 270.44,156.46
S$15899
  Bottom 0: 270.44,156.46 270.14,156.62
S$15900
  Bottom 0: 270.14,156.62 273.04,156.62
S$15901
  Bottom 0: 273.04,156.62 277.73,151.92
S$15902
  Bottom 0: 277.73,151.92 277.46,151.94
S$15903
  Bottom 0: 277.46,151.94 277.14,151.87
S$15904
  Bottom 0: 277.14,151.87 276.85,151.72
S$15905
  Bottom 0: 276.85,151.72 276.62,151.5
S$15906
  Bottom 0: 276.62,151.5 276.44,151.23
S$15907
  Bottom 0: 276.44,151.23 276.36,150.91
S$15908
  Bottom 0: 276.36,150.91 276.36,150.59
S$15909
  Bottom 0: 276.36,150.59 276.4,150.41
S$15910
  Bottom 0: 276.4,150.41 270.4,144.41
S$15911
  Bottom 0: 270.4,144.41 266.91,144.41
S$15912
  Bottom 0: 266.91,144.41 266.89,144.47
S$15913
  Bottom 0: 266.89,144.47 266.69,144.72
S$15914
  Bottom 0: 266.69,144.72 266.42,144.91
S$15915
  Bottom 0: 266.42,144.91 266.12,145.01
S$15916
  Bottom 0: 266.12,145.01 265.79,145.03
S$15917
  Bottom 0: 265.79,145.03 265.47,144.97
S$15918
  Bottom 0: 265.47,144.97 265.18,144.82
S$15919
  Bottom 0: 265.18,144.82 264.94,144.6
S$15920
  Bottom 0: 264.94,144.6 264.77,144.32
S$15921
  Bottom 0: 264.77,144.32 264.69,144.01
S$15922
  Bottom 0: 264.69,144.01 264.69,143.68
S$15923
  Bottom 0: 264.69,143.68 264.77,143.37
S$15924
  Bottom 0: 264.77,143.37 264.94,143.09
S$15925
  Bottom 0: 264.94,143.09 265.18,142.87
S$15926
  Bottom 0: 265.18,142.87 265.25,142.83
S$15927
  Bottom 0: 265.25,142.83 261.74,142.83
S$15928
  Bottom 0: 260.94,147.59 261.24,147.66
S$15929
  Bottom 0: 261.24,147.66 261.5,147.81
S$15930
  Bottom 0: 261.5,147.81 261.7,148.03
S$15931
  Bottom 0: 261.7,148.03 261.84,148.31
S$15932
  Bottom 0: 261.84,148.31 261.88,148.6
S$15933
  Bottom 0: 261.88,148.6 261.84,148.91
S$15934
  Bottom 0: 261.84,148.91 261.7,149.18
S$15935
  Bottom 0: 261.7,149.18 261.5,149.4
S$15936
  Bottom 0: 261.5,149.4 261.24,149.55
S$15937
  Bottom 0: 261.24,149.55 260.94,149.62
S$15938
  Bottom 0: 260.94,149.62 260.64,149.6
S$15939
  Bottom 0: 260.64,149.6 260.36,149.48
S$15940
  Bottom 0: 260.36,149.48 260.12,149.3
S$15941
  Bottom 0: 260.12,149.3 259.95,149.04
S$15942
  Bottom 0: 259.95,149.04 259.86,148.76
S$15943
  Bottom 0: 259.86,148.76 259.86,148.45
S$15944
  Bottom 0: 259.86,148.45 259.95,148.16
S$15945
  Bottom 0: 259.95,148.16 260.12,147.91
S$15946
  Bottom 0: 260.12,147.91 260.36,147.73
S$15947
  Bottom 0: 260.36,147.73 260.64,147.62
S$15948
  Bottom 0: 260.64,147.62 260.94,147.59
S$15949
  Bottom 0: 266.72,148.09 267.07,148.15
S$15950
  Bottom 0: 267.07,148.15 267.38,148.3
S$15951
  Bottom 0: 267.38,148.3 267.65,148.52
S$15952
  Bottom 0: 267.65,148.52 267.86,148.81
S$15953
  Bottom 0: 267.86,148.81 267.99,149.13
S$15954
  Bottom 0: 267.99,149.13 268.03,149.48
S$15955
  Bottom 0: 268.03,149.48 267.99,149.82
S$15956
  Bottom 0: 267.99,149.82 267.86,150.15
S$15957
  Bottom 0: 267.86,150.15 267.65,150.43
S$15958
  Bottom 0: 267.65,150.43 267.38,150.66
S$15959
  Bottom 0: 267.38,150.66 267.07,150.81
S$15960
  Bottom 0: 267.07,150.81 266.72,150.87
S$15961
  Bottom 0: 266.72,150.87 266.37,150.85
S$15962
  Bottom 0: 266.37,150.85 266.04,150.74
S$15963
  Bottom 0: 266.04,150.74 265.75,150.56
S$15964
  Bottom 0: 265.75,150.56 265.51,150.3
S$15965
  Bottom 0: 265.51,150.3 265.33,149.99
S$15966
  Bottom 0: 265.33,149.99 265.25,149.65
S$15967
  Bottom 0: 265.25,149.65 265.25,149.3
S$15968
  Bottom 0: 265.25,149.3 265.33,148.97
S$15969
  Bottom 0: 265.33,148.97 265.51,148.66
S$15970
  Bottom 0: 265.51,148.66 265.75,148.4
S$15971
  Bottom 0: 265.75,148.4 266.04,148.21
S$15972
  Bottom 0: 266.04,148.21 266.37,148.11
S$15973
  Bottom 0: 266.37,148.11 266.72,148.09
S$15974
  Bottom 0: 257.37,149.5 257.66,149.56
S$15975
  Bottom 0: 257.66,149.56 257.93,149.72
S$15976
  Bottom 0: 257.93,149.72 258.13,149.93
S$15977
  Bottom 0: 258.13,149.93 258.26,150.21
S$15978
  Bottom 0: 258.26,150.21 258.31,150.51
S$15979
  Bottom 0: 258.31,150.51 258.26,150.81
S$15980
  Bottom 0: 258.26,150.81 258.13,151.08
S$15981
  Bottom 0: 258.13,151.08 257.93,151.3
S$15982
  Bottom 0: 257.93,151.3 257.66,151.46
S$15983
  Bottom 0: 257.66,151.46 257.37,151.52
S$15984
  Bottom 0: 257.37,151.52 257.06,151.5
S$15985
  Bottom 0: 257.06,151.5 256.78,151.39
S$15986
  Bottom 0: 256.78,151.39 256.55,151.2
S$15987
  Bottom 0: 256.55,151.2 256.38,150.95
S$15988
  Bottom 0: 256.38,150.95 256.29,150.66
S$15989
  Bottom 0: 256.29,150.66 256.29,150.36
S$15990
  Bottom 0: 256.29,150.36 256.38,150.07
S$15991
  Bottom 0: 256.38,150.07 256.55,149.82
S$15992
  Bottom 0: 256.55,149.82 256.78,149.63
S$15993
  Bottom 0: 256.78,149.63 257.06,149.52
S$15994
  Bottom 0: 257.06,149.52 257.37,149.5
S$15995
  Bottom 0: 224.16,158.5 225.93,158.5
S$15996
  Bottom 0: 225.93,158.5 226.01,158.51
S$15997
  Bottom 0: 226.01,158.51 226.08,158.55
S$15998
  Bottom 0: 226.08,158.55 226.14,158.6
S$15999
  Bottom 0: 226.14,158.6 226.18,158.67
S$16000
  Bottom 0: 226.18,158.67 226.19,158.75
S$16001
  Bottom 0: 226.19,158.75 226.19,160.53
S$16002
  Bottom 0: 226.19,160.53 226.18,160.6
S$16003
  Bottom 0: 226.18,160.6 226.14,160.68
S$16004
  Bottom 0: 226.14,160.68 226.08,160.73
S$16005
  Bottom 0: 226.08,160.73 226.01,160.77
S$16006
  Bottom 0: 226.01,160.77 225.93,160.78
S$16007
  Bottom 0: 225.93,160.78 225.49,160.78
S$16008
  Bottom 0: 225.49,160.78 225.49,160.91
S$16009
  Bottom 0: 225.49,160.91 225.43,161.13
S$16010
  Bottom 0: 225.43,161.13 225.26,161.29
S$16011
  Bottom 0: 225.26,161.29 225.04,161.35
S$16012
  Bottom 0: 225.04,161.35 224.7,161.35
S$16013
  Bottom 0: 224.7,161.35 223.61,162.43
S$16014
  Bottom 0: 223.61,162.43 223.67,162.57
S$16015
  Bottom 0: 223.67,162.57 223.72,162.89
S$16016
  Bottom 0: 223.72,162.89 223.67,163.22
S$16017
  Bottom 0: 223.67,163.22 223.54,163.51
S$16018
  Bottom 0: 223.54,163.51 223.34,163.77
S$16019
  Bottom 0: 223.34,163.77 223.07,163.96
S$16020
  Bottom 0: 223.07,163.96 222.77,164.06
S$16021
  Bottom 0: 222.77,164.06 222.44,164.08
S$16022
  Bottom 0: 222.44,164.08 222.12,164.02
S$16023
  Bottom 0: 222.12,164.02 221.83,163.87
S$16024
  Bottom 0: 221.83,163.87 221.6,163.65
S$16025
  Bottom 0: 221.6,163.65 221.43,163.37
S$16026
  Bottom 0: 221.43,163.37 221.34,163.06
S$16027
  Bottom 0: 221.34,163.06 221.34,162.73
S$16028
  Bottom 0: 221.34,162.73 221.43,162.42
S$16029
  Bottom 0: 221.43,162.42 221.6,162.14
S$16030
  Bottom 0: 221.6,162.14 221.83,161.92
S$16031
  Bottom 0: 221.83,161.92 222.12,161.77
S$16032
  Bottom 0: 222.12,161.77 222.44,161.71
S$16033
  Bottom 0: 222.44,161.71 222.77,161.73
S$16034
  Bottom 0: 222.77,161.73 222.99,161.8
S$16035
  Bottom 0: 222.99,161.8 224.05,160.75
S$16036
  Bottom 0: 224.05,160.75 224.01,160.73
S$16037
  Bottom 0: 224.01,160.73 223.95,160.68
S$16038
  Bottom 0: 223.95,160.68 223.91,160.6
S$16039
  Bottom 0: 223.91,160.6 223.9,160.53
S$16040
  Bottom 0: 223.9,160.53 223.9,158.75
S$16041
  Bottom 0: 223.9,158.75 223.91,158.67
S$16042
  Bottom 0: 223.91,158.67 223.95,158.6
S$16043
  Bottom 0: 223.95,158.6 224.01,158.55
S$16044
  Bottom 0: 224.01,158.55 224.08,158.51
S$16045
  Bottom 0: 224.08,158.51 224.16,158.5
S$16046
  Bottom 0: 220.54,164.08 220.86,164.1
S$16047
  Bottom 0: 220.86,164.1 221.17,164.21
S$16048
  Bottom 0: 221.17,164.21 221.43,164.39
S$16049
  Bottom 0: 221.43,164.39 221.64,164.65
S$16050
  Bottom 0: 221.64,164.65 221.76,164.95
S$16051
  Bottom 0: 221.76,164.95 221.81,165.27
S$16052
  Bottom 0: 221.81,165.27 221.76,165.59
S$16053
  Bottom 0: 221.76,165.59 221.64,165.89
S$16054
  Bottom 0: 221.64,165.89 221.43,166.14
S$16055
  Bottom 0: 221.43,166.14 221.17,166.33
S$16056
  Bottom 0: 221.17,166.33 220.86,166.44
S$16057
  Bottom 0: 220.86,166.44 220.54,166.46
S$16058
  Bottom 0: 220.54,166.46 220.22,166.39
S$16059
  Bottom 0: 220.22,166.39 219.93,166.24
S$16060
  Bottom 0: 219.93,166.24 219.69,166.02
S$16061
  Bottom 0: 219.69,166.02 219.52,165.75
S$16062
  Bottom 0: 219.52,165.75 219.44,165.43
S$16063
  Bottom 0: 219.44,165.43 219.44,165.1
S$16064
  Bottom 0: 219.44,165.1 219.52,164.79
S$16065
  Bottom 0: 219.52,164.79 219.69,164.52
S$16066
  Bottom 0: 219.69,164.52 219.93,164.29
S$16067
  Bottom 0: 219.93,164.29 220.22,164.15
S$16068
  Bottom 0: 220.22,164.15 220.54,164.08
S$16069
  Bottom 0: 40.87,144.67 33.06,152.47
S$16070
  Bottom 0: 33.06,152.47 33.01,152.52
S$16071
  Bottom 0: 33.01,152.52 32.94,152.56
S$16072
  Bottom 0: 32.94,152.56 32.88,152.58
S$16073
  Bottom 0: 32.88,152.58 32.81,152.6
S$16074
  Bottom 0: 32.81,152.6 32.75,152.6
S$16075
  Bottom 0: 32.75,152.6 31.23,152.6
S$16076
  Bottom 0: 31.23,152.6 31.23,153.03
S$16077
  Bottom 0: 31.23,153.03 31.23,153.11
S$16078
  Bottom 0: 31.23,153.11 31.21,153.17
S$16079
  Bottom 0: 31.21,153.17 31.18,153.23
S$16080
  Bottom 0: 31.18,153.23 31.14,153.29
S$16081
  Bottom 0: 31.14,153.29 31.1,153.35
S$16082
  Bottom 0: 31.1,153.35 30.64,153.82
S$16083
  Bottom 0: 30.64,153.82 30.58,153.86
S$16084
  Bottom 0: 30.58,153.86 30.52,153.9
S$16085
  Bottom 0: 30.52,153.9 30.46,153.92
S$16086
  Bottom 0: 30.46,153.92 30.39,153.94
S$16087
  Bottom 0: 30.39,153.94 30.32,153.94
S$16088
  Bottom 0: 30.32,153.94 29.82,153.94
S$16089
  Bottom 0: 29.82,153.94 26.16,157.61
S$16090
  Bottom 0: 26.16,157.61 26.36,157.6
S$16091
  Bottom 0: 26.36,157.6 26.66,157.66
S$16092
  Bottom 0: 26.66,157.66 26.92,157.81
S$16093
  Bottom 0: 26.92,157.81 26.93,157.82
S$16094
  Bottom 0: 26.93,157.82 37.66,157.82
S$16095
  Bottom 0: 37.66,157.82 37.73,157.83
S$16096
  Bottom 0: 37.73,157.83 37.8,157.85
S$16097
  Bottom 0: 37.8,157.85 37.86,157.87
S$16098
  Bottom 0: 37.86,157.87 37.92,157.91
S$16099
  Bottom 0: 37.92,157.91 37.98,157.95
S$16100
  Bottom 0: 37.98,157.95 39.32,159.29
S$16101
  Bottom 0: 39.32,159.29 44.59,159.29
S$16102
  Bottom 0: 44.59,159.29 44.42,159.04
S$16103
  Bottom 0: 44.42,159.04 44.33,158.75
S$16104
  Bottom 0: 44.33,158.75 44.33,158.45
S$16105
  Bottom 0: 44.33,158.45 44.42,158.16
S$16106
  Bottom 0: 44.42,158.16 44.59,157.91
S$16107
  Bottom 0: 44.59,157.91 44.83,157.72
S$16108
  Bottom 0: 44.83,157.72 45.11,157.61
S$16109
  Bottom 0: 45.11,157.61 45.41,157.59
S$16110
  Bottom 0: 45.41,157.59 45.66,157.65
S$16111
  Bottom 0: 45.66,157.65 45.88,157.42
S$16112
  Bottom 0: 45.88,157.42 45.9,157.41
S$16113
  Bottom 0: 45.9,157.41 44.57,157.41
S$16114
  Bottom 0: 44.57,157.41 44.5,157.41
S$16115
  Bottom 0: 44.5,157.41 44.44,157.39
S$16116
  Bottom 0: 44.44,157.39 44.37,157.37
S$16117
  Bottom 0: 44.37,157.37 44.31,157.33
S$16118
  Bottom 0: 44.31,157.33 44.26,157.28
S$16119
  Bottom 0: 44.26,157.28 40.24,153.26
S$16120
  Bottom 0: 40.24,153.26 40.06,153.35
S$16121
  Bottom 0: 40.06,153.35 39.71,153.41
S$16122
  Bottom 0: 39.71,153.41 39.36,153.39
S$16123
  Bottom 0: 39.36,153.39 39.03,153.28
S$16124
  Bottom 0: 39.03,153.28 38.73,153.1
S$16125
  Bottom 0: 38.73,153.1 38.49,152.84
S$16126
  Bottom 0: 38.49,152.84 38.32,152.53
S$16127
  Bottom 0: 38.32,152.53 38.23,152.19
S$16128
  Bottom 0: 38.23,152.19 38.23,151.84
S$16129
  Bottom 0: 38.23,151.84 38.32,151.51
S$16130
  Bottom 0: 38.32,151.51 38.49,151.2
S$16131
  Bottom 0: 38.49,151.2 38.73,150.94
S$16132
  Bottom 0: 38.73,150.94 39.03,150.75
S$16133
  Bottom 0: 39.03,150.75 39.36,150.65
S$16134
  Bottom 0: 39.36,150.65 39.71,150.63
S$16135
  Bottom 0: 39.71,150.63 40.06,150.69
S$16136
  Bottom 0: 40.06,150.69 40.37,150.84
S$16137
  Bottom 0: 40.37,150.84 40.64,151.06
S$16138
  Bottom 0: 40.64,151.06 40.85,151.35
S$16139
  Bottom 0: 40.85,151.35 40.98,151.67
S$16140
  Bottom 0: 40.98,151.67 41.02,152.02
S$16141
  Bottom 0: 41.02,152.02 40.98,152.36
S$16142
  Bottom 0: 40.98,152.36 40.87,152.64
S$16143
  Bottom 0: 40.87,152.64 44.76,156.53
S$16144
  Bottom 0: 44.76,156.53 53.73,156.53
S$16145
  Bottom 0: 53.73,156.53 53.59,156.46
S$16146
  Bottom 0: 53.59,156.46 53.25,156.17
S$16147
  Bottom 0: 53.25,156.17 52.96,155.83
S$16148
  Bottom 0: 52.96,155.83 52.75,155.43
S$16149
  Bottom 0: 52.75,155.43 52.62,155.01
S$16150
  Bottom 0: 52.62,155.01 52.58,154.56
S$16151
  Bottom 0: 52.58,154.56 52.62,154.11
S$16152
  Bottom 0: 52.62,154.11 52.75,153.68
S$16153
  Bottom 0: 52.75,153.68 52.96,153.29
S$16154
  Bottom 0: 52.96,153.29 53.25,152.94
S$16155
  Bottom 0: 53.25,152.94 53.59,152.66
S$16156
  Bottom 0: 53.59,152.66 53.99,152.45
S$16157
  Bottom 0: 53.99,152.45 54.42,152.32
S$16158
  Bottom 0: 54.42,152.32 54.86,152.27
S$16159
  Bottom 0: 54.86,152.27 55.31,152.32
S$16160
  Bottom 0: 55.31,152.32 55.74,152.45
S$16161
  Bottom 0: 55.74,152.45 56.13,152.66
S$16162
  Bottom 0: 56.13,152.66 56.48,152.94
S$16163
  Bottom 0: 56.48,152.94 56.76,153.29
S$16164
  Bottom 0: 56.76,153.29 56.98,153.68
S$16165
  Bottom 0: 56.98,153.68 57.1,154.11
S$16166
  Bottom 0: 57.1,154.11 57.15,154.56
S$16167
  Bottom 0: 57.15,154.56 57.1,155.01
S$16168
  Bottom 0: 57.1,155.01 56.98,155.43
S$16169
  Bottom 0: 56.98,155.43 56.76,155.83
S$16170
  Bottom 0: 56.76,155.83 56.48,156.17
S$16171
  Bottom 0: 56.48,156.17 56.13,156.46
S$16172
  Bottom 0: 56.13,156.46 56,156.53
S$16173
  Bottom 0: 56,156.53 72.78,156.53
S$16174
  Bottom 0: 72.78,156.53 72.64,156.46
S$16175
  Bottom 0: 72.64,156.46 72.3,156.17
S$16176
  Bottom 0: 72.3,156.17 72.01,155.83
S$16177
  Bottom 0: 72.01,155.83 71.8,155.43
S$16178
  Bottom 0: 71.8,155.43 71.67,155.01
S$16179
  Bottom 0: 71.67,155.01 71.63,154.56
S$16180
  Bottom 0: 71.63,154.56 71.67,154.11
S$16181
  Bottom 0: 71.67,154.11 71.8,153.68
S$16182
  Bottom 0: 71.8,153.68 72.01,153.29
S$16183
  Bottom 0: 72.01,153.29 72.3,152.94
S$16184
  Bottom 0: 72.3,152.94 72.64,152.66
S$16185
  Bottom 0: 72.64,152.66 73.04,152.45
S$16186
  Bottom 0: 73.04,152.45 73.47,152.32
S$16187
  Bottom 0: 73.47,152.32 73.91,152.27
S$16188
  Bottom 0: 73.91,152.27 74.36,152.32
S$16189
  Bottom 0: 74.36,152.32 74.79,152.45
S$16190
  Bottom 0: 74.79,152.45 75.18,152.66
S$16191
  Bottom 0: 75.18,152.66 75.53,152.94
S$16192
  Bottom 0: 75.53,152.94 75.81,153.29
S$16193
  Bottom 0: 75.81,153.29 76.03,153.68
S$16194
  Bottom 0: 76.03,153.68 76.15,154.11
S$16195
  Bottom 0: 76.15,154.11 76.2,154.56
S$16196
  Bottom 0: 76.2,154.56 76.15,155.01
S$16197
  Bottom 0: 76.15,155.01 76.12,155.13
S$16198
  Bottom 0: 76.12,155.13 77.84,153.41
S$16199
  Bottom 0: 77.84,153.41 77.81,153.41
S$16200
  Bottom 0: 77.81,153.41 77.46,153.39
S$16201
  Bottom 0: 77.46,153.39 77.13,153.28
S$16202
  Bottom 0: 77.13,153.28 76.83,153.1
S$16203
  Bottom 0: 76.83,153.1 76.59,152.84
S$16204
  Bottom 0: 76.59,152.84 76.42,152.53
S$16205
  Bottom 0: 76.42,152.53 76.33,152.19
S$16206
